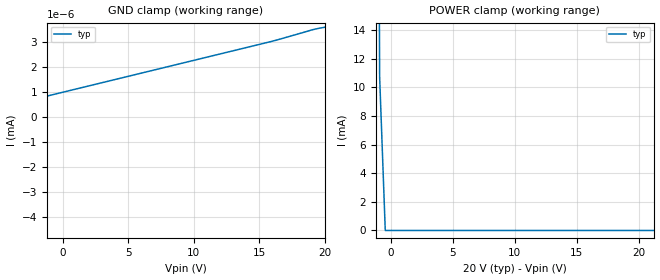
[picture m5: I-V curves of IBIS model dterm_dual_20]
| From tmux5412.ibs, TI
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| dterm_dual_20
[Model]   dterm_dual_20
Model_type   Terminator
|   typ   min   max
C_comp   1.008417e-11   NA   NA
[Voltage Range]   20   NA   NA
[Temperature Range]   27   NA   NA
[Power Clamp Reference]   20   NA   NA
[GND Clamp Reference]   0   NA   NA
[GND Clamp]
|   Voltage   I(typ)   I(min)   I(max)
-25V      -2.839A    NA         NA
-20.45V   -1.081uA   NA         NA
-20V      -1.588nA   NA         NA
-15.91V   -1.034nA   NA         NA
15.91V    3.008nA    NA         NA
19.09V    3.479nA    NA         NA
20V       3.577nA    NA         NA
[POWER Clamp]
|   Voltage   I(typ)   I(min)   I(max)
-5V       2.61A      NA         NA
-1.364V   106.7mA    NA         NA
-909.1mV  10.75mA    NA         NA
-454.5mV  126.5nA    NA         NA
40V       -1.588nA   NA         NA
